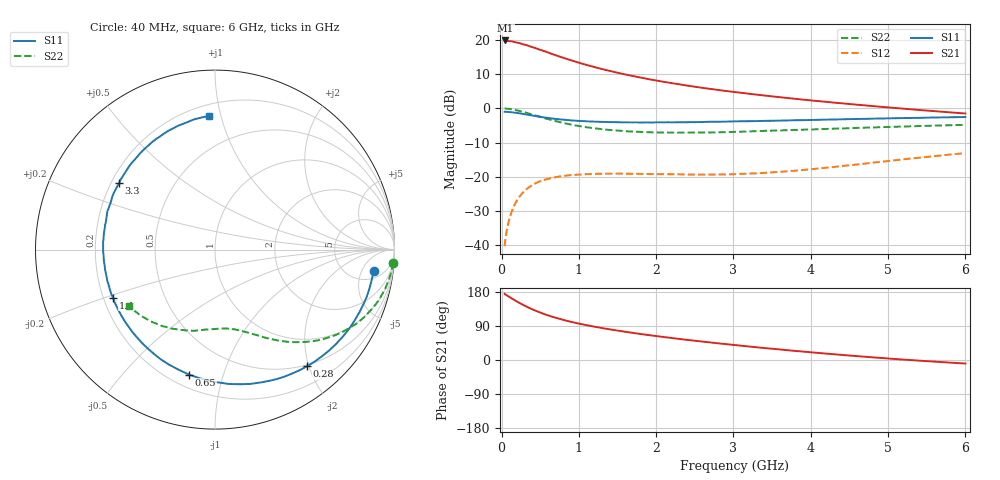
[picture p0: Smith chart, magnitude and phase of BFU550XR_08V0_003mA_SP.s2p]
! Filename:  P:\Prog\Test\Noise\ATS_data\Testdata_Net\03 Spar\BFU550XR_APG2013_45_C05_08p0V_003mA_SP_CM01_D.s2p
! Date/Time: Tue 06/Aug/2013 14:38:17
! BFU550XR_APG2013_45_C05_08p0V_1to35mA_SP_CM01_Bias3_R.s2p
! MDIF S-parameter v. bias file
! BFU550XR_APG2013_45_C05_08p0V_1to35mA_SP_CM01
! Date/time Fri Aug 02 14:53:20 2013
! VAR V_out= 8.0010
! VAR I_out= 3.0000
! VAR V_in= 0.7981
! VAR I_in= 0.0315
! Device data file deembeded for feedlines and parallel
! Original file: \03 Spar\BFU550XR_APG2013_45_C05_08p0V_003mA_SP_CM01_R.s2p
! Feed-files: PR006V01_02082013_Feed1.s2p, PR006V01_02082013_Feed2.s2p
! Parallel-file: PR006V01_02082013_Par.s2p
# MHz S MA R 50
!  Freq-MHz  S11-mag  S11-arg  S21-mag  S21-arg  S12-mag  S12-arg  S22-mag  S22-arg
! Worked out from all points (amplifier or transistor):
!   98 points, 40 MHz to 6 GHz, reference 50 ohm
!   highest |S21| = 19.8 dB at 50 MHz (marker M1)
!   |S21| within 3 dB of that: start of sweep to 536.1 MHz
!   unconditionally stable (mu >= 1): 2.779 GHz to 4.43 GHz
!   at 300 MHz: K = 0.12, MSG = 21.4 dB, |S12| = -24.1 dB
!   at 1.6 GHz: K = 0.61, MSG = 14.5 dB, |S12| = -19.1 dB
!   at 6 GHz: K = 0.81, MSG = 5.8 dB, |S12| = -13.1 dB
!   S11 on the Smith chart (normalised r, x): 40 MHz: 7, -9; 280 MHz: 0.48, -1.97; 650 MHz: 0.28, -0.78; 1.4 GHz: 0.24, -0.21; 3.3 GHz: 0.23, +0.30; 6 GHz: 0.27, +0.92
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40  0.8915 -7.8  9.81 174.5  0.009661 85.0  0.9946 -4.2
50  0.8905 -9.8  9.813 172.6  0.01206 84.3  0.9933 -5.3
120  0.8774 -23.3  9.579 163.9  0.02827 76.5  0.9735 -12.9
180  0.8613 -34.4  9.224 156.6  0.0411 70.3  0.9453 -18.9
240  0.8412 -45.1  8.929 149.7  0.05244 64.7  0.9118 -24.5
280  0.8281 -51.6  8.601 145.4  0.05925 61.1  0.8872 -27.9
320  0.812 -58.6  8.422 141.1  0.06532 57.8  0.8605 -31.1
440  0.7702 -76.4  7.577 130.1  0.08018 49.3  0.7851 -39.3
550  0.7361 -90.7  6.864 121.3  0.08965 42.9  0.7202 -45.6
650  0.7116 -101.7  6.242 114.6  0.09622 38.3  0.6724 -50.0
850  0.6732 -120.4  5.243 103.2  0.1043 31.3  0.594 -57.3
1050  0.6502 -135.0  4.47 94.0  0.1081 26.5  0.5389 -63.0
1200  0.6388 -144.2  4.012 88.0  0.1099 23.9  0.5107 -66.5
1400  0.6286 -154.8  3.52 80.9  0.1108 21.3  0.4829 -70.8
1700  0.6222 -167.9  2.964 71.5  0.1103 19.3  0.4565 -76.5
2050  0.6233 179.7  2.491 61.9  0.1089 18.8  0.4429 -82.7
2500  0.6272 165.8  2.067 50.8  0.1076 20.3  0.4425 -90.2
3100  0.6468 150.0  1.686 37.7  0.11 26.0  0.4553 -100.0
3300  0.6507 145.3  1.584 33.5  0.1122 28.0  0.4643 -103.4
4100  0.6799 127.8  1.274 18.6  0.1321 35.3  0.4948 -116.5
5200  0.7204 106.4  0.9883 1.1  0.1798 37.4  0.5417 -134.1
6000  0.7462 92.5  0.8397 -9.3  0.2212 33.8  0.5735 -146.7
